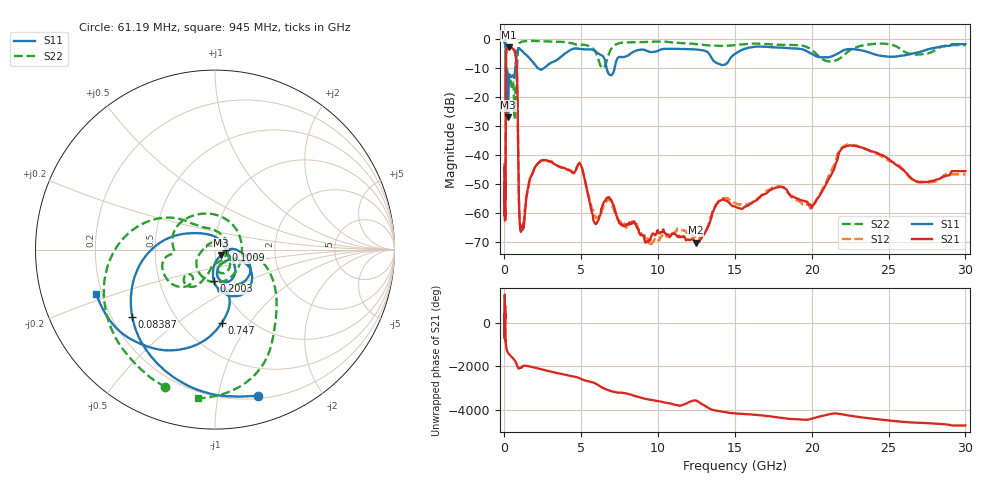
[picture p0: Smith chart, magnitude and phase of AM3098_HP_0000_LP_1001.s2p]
! Date/Time: Thu, Feb 28, 2019 8:30 AM
! Network Analyzer: Agilent Technologies E8364B Rev: A.07.50.67
! Sweep from 0.010 to 30.000 GHz, 1601 Points, Sweep Type: LOG
! Power Supply: 5.023 V, 0.002 A
# Hz S DB R 50
!freq MagS11 AngS11 MagS21 AngS21 MagS12 AngS12 MagS22 AngS22
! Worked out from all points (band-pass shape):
!   1601 points, 10 MHz to 30 GHz, reference 50 ohm
!   highest |S21| = -2.77 dB at 265.1 MHz (marker M1); lowest = -70.3 dB at 12.43 GHz (marker M2)
!   |S21| within 3 dB of the highest: 104.6 MHz to 734.9 MHz (630.3 MHz wide, 150 % of centre)
!   lowest |S11| = -26.9 dB at 232.8 MHz (marker M3), VSWR 1.09, Z = 53.2 - j3.36 ohm
!   |S11| at or under -10 dB: 90.38 MHz to 701.6 MHz (611.2 MHz wide, 154 % of centre); 2.189 GHz to 2.548 GHz (358.5 MHz wide, 15.1 % of centre); 6.647 GHz to 7.168 GHz (520.8 MHz wide, 7.54 % of centre)
!   |S22| runs from -27.5 to -0.5 dB; largest |S21 - S12| = 0.012
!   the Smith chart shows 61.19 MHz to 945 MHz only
!   S11 on the Smith chart (normalised r, x): 61.19 MHz: 0.23, -1.31; 83.87 MHz: 0.28, -0.33; 100.9 MHz: 1.13, -0.01; 200.3 MHz: 0.93, -0.34; 747 MHz: 0.76, -0.75; 945 MHz: 0.18, -0.17
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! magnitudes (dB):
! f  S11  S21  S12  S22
! 10 MHz  -0.4  -44.7  -44.0  -0.6
! 38.04 MHz  -0.5  -60.8  -60.8  -1.0
! 61.19 MHz  -1.4  -51.2  -54.3  -1.8
! 70.4 MHz  -2.0  -52.3  -52.2  -2.4
! 83.87 MHz  -4.5  -28.5  -28.4  -5.0
! 100.9 MHz  -24.1  -6.6  -6.6  -16.5
! 144.7 MHz  -14.5  -3.4  -3.4  -12.7
! 200.3 MHz  -15.0  -3.1  -3.0  -10.9
! 232.8 MHz  -26.9  -2.8  -2.8  -12.5
! 265.1 MHz  -17.6  -2.8  -2.7  -12.8
! 550.5 MHz  -12.5  -3.3  -3.3  -14.7
! 747 MHz  -7.7  -6.3  -6.2  -21.1
! 833.9 MHz  -4.2  -16.0  -15.9  -7.6
! 945 MHz  -3.0  -56.3  -56.1  -1.6
! 1.226 GHz  -4.4  -64.8  -64.5  -0.7
! 2.084 GHz  -9.4  -43.5  -43.6  -0.6
! 4.903 GHz  -3.3  -42.9  -42.6  -1.9
! 7.926 GHz  -5.9  -64.0  -65.1  -1.0
! 12.43 GHz  -3.5  -70.3  -68.6  -1.6
! 19.9 GHz  -4.7  -57.0  -58.4  -3.2
! 22.56 GHz  -3.3  -36.6  -36.4  -3.5
! 30 GHz  -1.7  -45.5  -46.6  -2.0
